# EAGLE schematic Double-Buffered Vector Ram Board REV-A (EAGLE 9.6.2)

## Sheet 1 of 4: Vector Ram Control
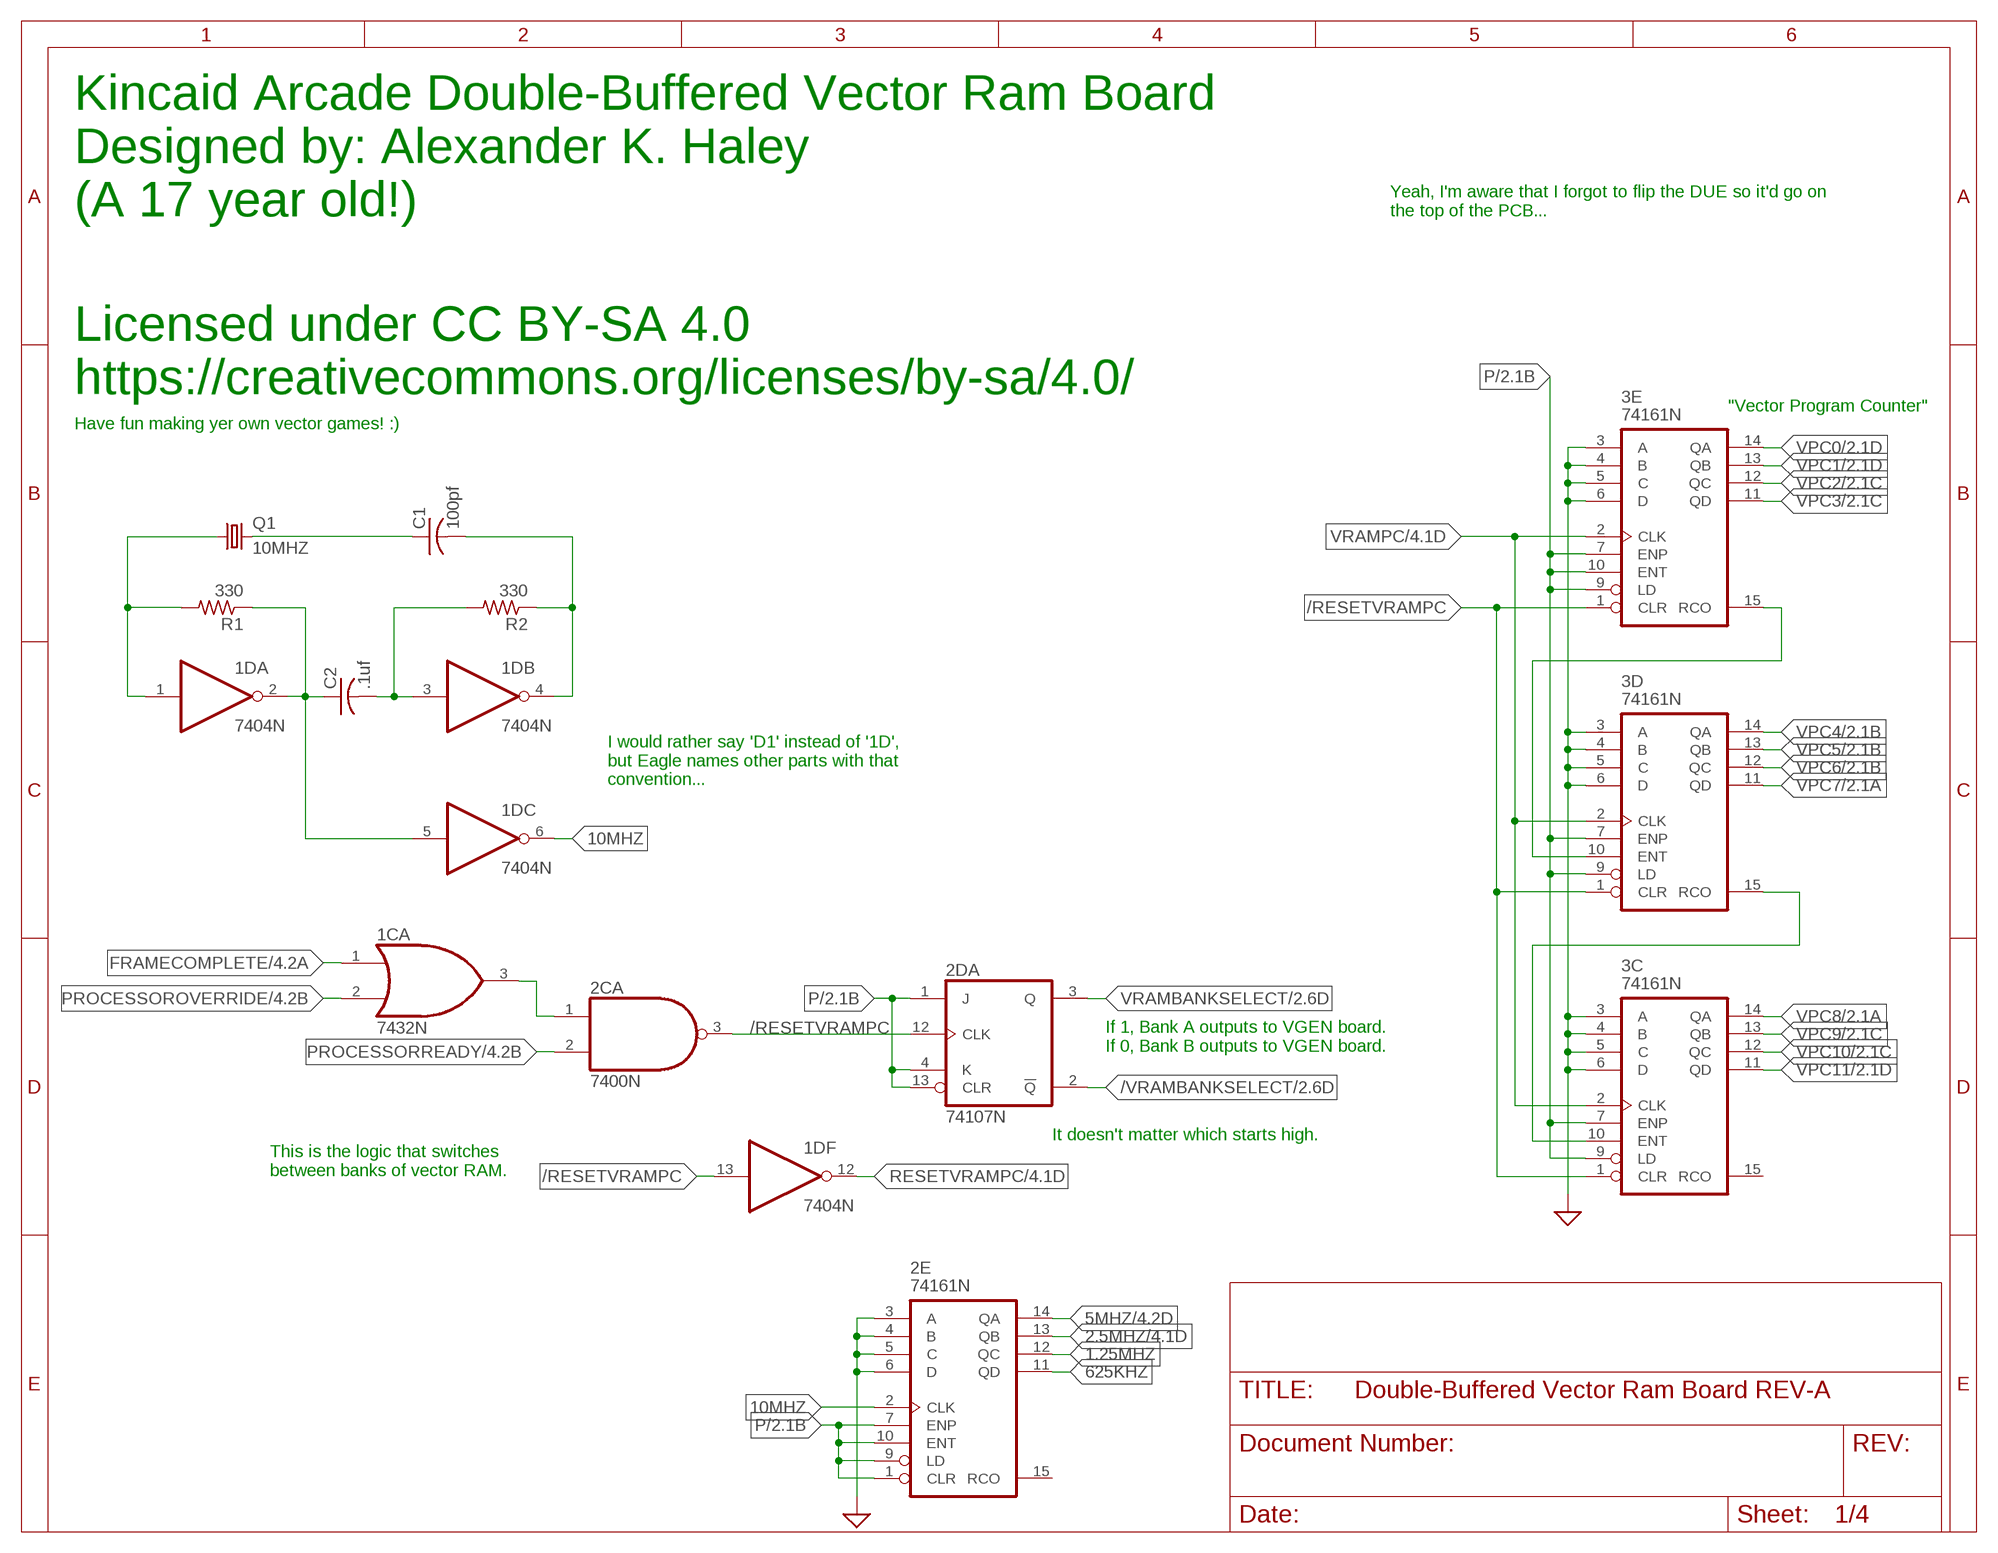
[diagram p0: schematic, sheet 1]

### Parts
1C  7432N  [DIL14]
1D  7404N  [DIL14]
2C  7400N  [DIL14]
2D  74107N  [DIL14]
2E  74161N  [DIL16]
3C  74161N  [DIL16]
3D  74161N  [DIL16]
3E  74161N  [DIL16]
C1  100pf  C-US025-030X050  [C025-030X050]
C2  .1uf  C-US050-050X075  [C050-050X075]
Q1  10MHZ  CRYSTALHC49S  [HC49/S]
R1  330  R-US_0207/10  [0207/10]
R2  330  R-US_0207/10  [0207/10]

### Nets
1.25MHZ: 2E.12(QC)
2.5MHZ: 2E.13(QB) ; also sheet 4
5MHZ: 2E.14(QA) ; also sheet 4
10MHZ: 1D.6(C:O) 2E.2(CLK)
625KHZ: 2E.11(QD)
/RESETVRAMPC: 1D.13(F:I) 2C.3(A:O) 2D.12(A:CLK) 3C.1(CLR) 3D.1(CLR) 3E.1(CLR)
/VRAMBANKSELECT: 2D.2(A:!Q) ; also sheet 2,3
FRAMECOMPLETE: 1C.1(A:I0) ; also sheet 4
GND: 2E.3(A) 2E.4(B) 2E.5(C) 2E.6(D) 3C.3(A) 3C.4(B) 3C.5(C) 3C.6(D) 3D.3(A) 3D.4(B) 3D.5(C) 3D.6(D) 3E.3(A) 3E.4(B) 3E.5(C) 3E.6(D) ; supply symbol labelled SUP ; also sheet 2,3,4
N$2: 1C.3(A:O) 2C.1(A:I0)
N$5: 3C.10(ENT) 3D.15(RCO)
N$6: 3D.10(ENT) 3E.15(RCO)
N$48: 1D.1(A:I) Q1.1 R1.2
N$52: 1D.2(A:O) 1D.5(C:I) C2.1 R1.1
N$61: 1D.3(B:I) C2.2 R2.2
N$69: C1.1 Q1.2
N$74: 1D.4(B:O) C1.2 R2.1
P: 2D.1(A:J) 2D.4(A:K) 2D.13(A:CLR) 2E.1(CLR) 2E.7(ENP) 2E.9(LD) 2E.10(ENT) 3C.7(ENP) 3C.9(LD) 3D.7(ENP) 3D.9(LD) 3E.7(ENP) 3E.9(LD) 3E.10(ENT) ; also sheet 2,3,4
PROCESSOROVERRIDE: 1C.2(A:I1) ; also sheet 4
PROCESSORREADY: 2C.2(A:I1) ; also sheet 4
RESETVRAMPC: 1D.12(F:O) ; also sheet 4
VPC0: 3E.14(QA) ; also sheet 2,3
VPC1: 3E.13(QB) ; also sheet 2,3
VPC2: 3E.12(QC) ; also sheet 2,3
VPC3: 3E.11(QD) ; also sheet 2,3
VPC4: 3D.14(QA) ; also sheet 2,3
VPC5: 3D.13(QB) ; also sheet 2,3
VPC6: 3D.12(QC) ; also sheet 2,3
VPC7: 3D.11(QD) ; also sheet 2,3
VPC8: 3C.14(QA) ; also sheet 2,3
VPC9: 3C.13(QB) ; also sheet 2,3
VPC10: 3C.12(QC) ; also sheet 2,3
VPC11: 3C.11(QD) ; also sheet 2,3
VRAMBANKSELECT: 2D.3(A:Q) ; also sheet 2,3
VRAMPC: 3C.2(CLK) 3D.2(CLK) 3E.2(CLK) ; also sheet 4
Unconnected: 2E.15(RCO) 3C.15(RCO)

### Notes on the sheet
- Kincaid Arcade Double-Buffered Vector Ram Board
- Designed by: Alexander K. Haley
- (A 17 year old!)
- Yeah, I'm aware that I forgot to flip the DUE so it'd go on
  the top of the PCB...
- Licensed under CC BY-SA 4.0
- https://creativecommons.org/licenses/by-sa/4.0/
- "Vector Program Counter"
- Have fun making yer own vector games! :)
- I would rather say 'D1' instead of '1D',
  but Eagle names other parts with that
  convention...
- If 1, Bank A outputs to VGEN board.
  If 0, Bank B outputs to VGEN board.
- It doesn't matter which starts high.
- This is the logic that switches 
  between banks of vector RAM.

## Sheet 2 of 4: Vector Ram Bank A
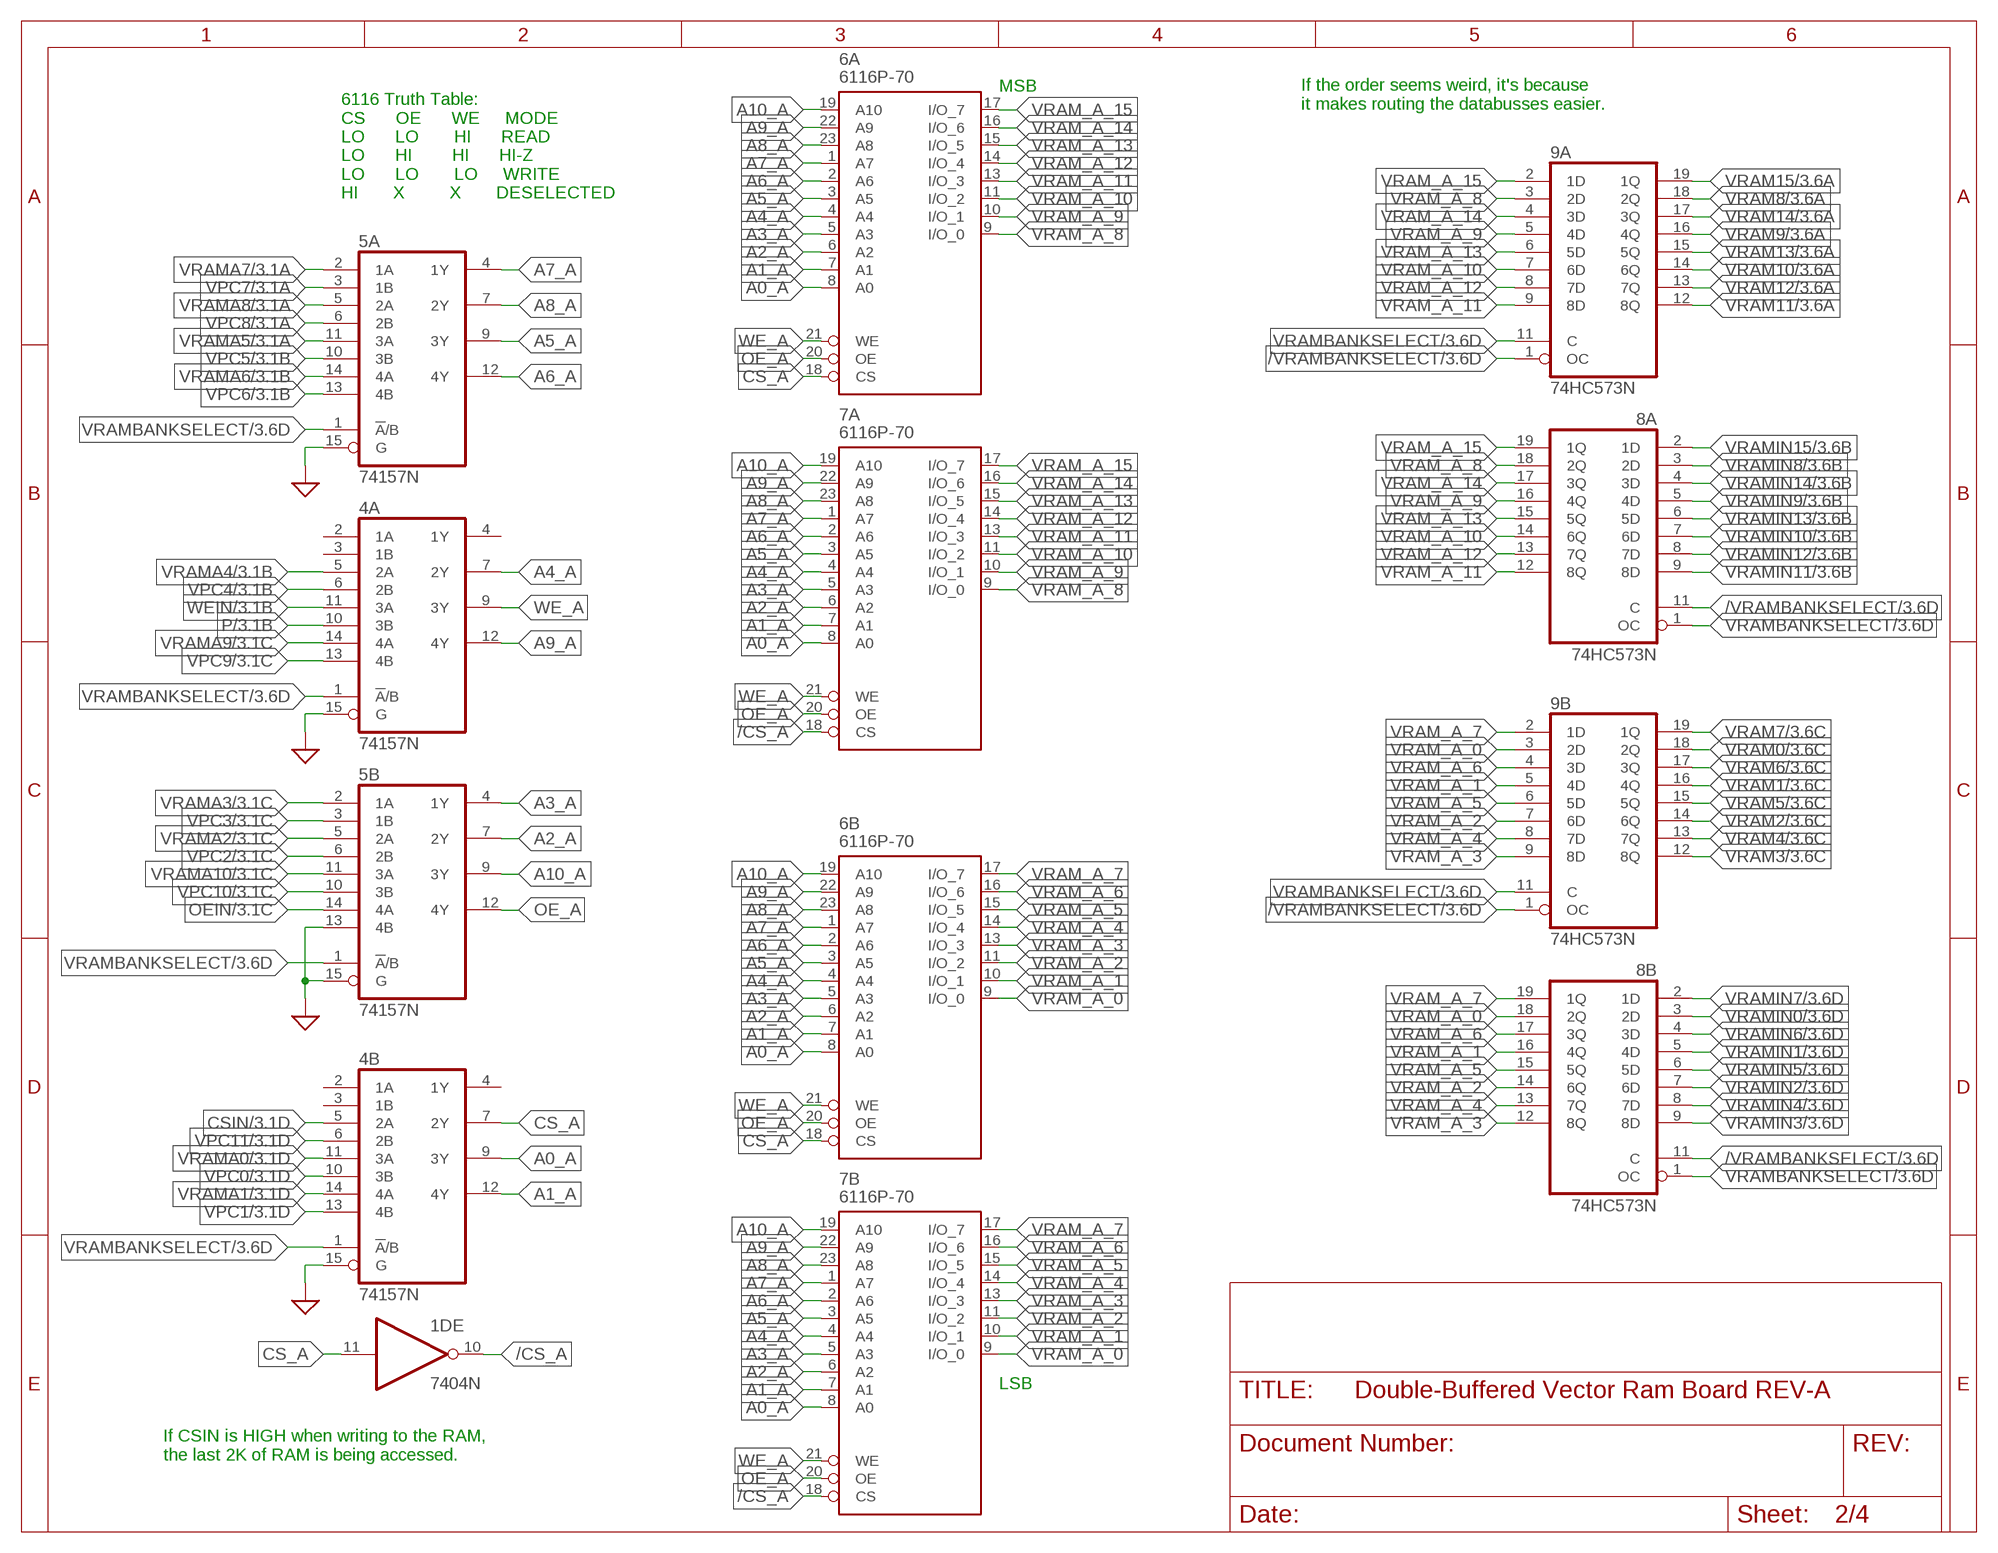
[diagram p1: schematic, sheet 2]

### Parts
4A  74157N  [DIL16]
4B  74157N  [DIL16]
5A  74157N  [DIL16]
5B  74157N  [DIL16]
6A  6116P-70  [DIL24]
6B  6116P-70  [DIL24]
7A  6116P-70  DS1220AB/AD  [DIL24]
7B  6116P-70  DS1220AB/AD  [DIL24]
8A  74HC573N  [DIL20]
8B  74HC573N  [DIL20]
9A  74HC573N  [DIL20]
9B  74HC573N  [DIL20]

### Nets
/CS_A: 1D.10(E:O) 7A.18(CS) 7B.18(CS)
/VRAMBANKSELECT: 8A.11(C) 8B.11(C) 9A.1(OC) 9B.1(OC) ; also sheet 1,3
A0_A: 4B.9(3Y) 6A.8(A0) 6B.8(A0) 7A.8(A0) 7B.8(A0)
A1_A: 4B.12(4Y) 6A.7(A1) 6B.7(A1) 7A.7(A1) 7B.7(A1)
A2_A: 5B.7(2Y) 6A.6(A2) 6B.6(A2) 7A.6(A2) 7B.6(A2)
A3_A: 5B.4(1Y) 6A.5(A3) 6B.5(A3) 7A.5(A3) 7B.5(A3)
A4_A: 4A.7(2Y) 6A.4(A4) 6B.4(A4) 7A.4(A4) 7B.4(A4)
A5_A: 5A.9(3Y) 6A.3(A5) 6B.3(A5) 7A.3(A5) 7B.3(A5)
A6_A: 5A.12(4Y) 6A.2(A6) 6B.2(A6) 7A.2(A6) 7B.2(A6)
A7_A: 5A.4(1Y) 6A.1(A7) 6B.1(A7) 7A.1(A7) 7B.1(A7)
A8_A: 5A.7(2Y) 6A.23(A8) 6B.23(A8) 7A.23(A8) 7B.23(A8)
A9_A: 4A.12(4Y) 6A.22(A9) 6B.22(A9) 7A.22(A9) 7B.22(A9)
A10_A: 5B.9(3Y) 6A.19(A10) 6B.19(A10) 7A.19(A10) 7B.19(A10)
CS_A: 1D.11(E:I) 4B.7(2Y) 6A.18(CS) 6B.18(CS)
CSIN: 4B.5(2A) ; also sheet 3,4
GND: 4A.15(G) 4B.15(G) 5A.15(G) 5B.13(4B) 5B.15(G) ; supply symbol labelled SUP ; also sheet 1,3,4
OE_A: 5B.12(4Y) 6A.20(OE) 6B.20(OE) 7A.20(OE) 7B.20(OE)
OEIN: 5B.14(4A) ; also sheet 3,4
P: 4A.10(3B) ; also sheet 1,3,4
VPC0: 4B.10(3B) ; also sheet 1,3
VPC1: 4B.13(4B) ; also sheet 1,3
VPC2: 5B.6(2B) ; also sheet 1,3
VPC3: 5B.3(1B) ; also sheet 1,3
VPC4: 4A.6(2B) ; also sheet 1,3
VPC5: 5A.10(3B) ; also sheet 1,3
VPC6: 5A.13(4B) ; also sheet 1,3
VPC7: 5A.3(1B) ; also sheet 1,3
VPC8: 5A.6(2B) ; also sheet 1,3
VPC9: 4A.13(4B) ; also sheet 1,3
VPC10: 5B.10(3B) ; also sheet 1,3
VPC11: 4B.6(2B) ; also sheet 1,3
VRAM0: 9B.18(2Q) ; also sheet 3,4
VRAM1: 9B.16(4Q) ; also sheet 3,4
VRAM2: 9B.14(6Q) ; also sheet 3,4
VRAM3: 9B.12(8Q) ; also sheet 3,4
VRAM4: 9B.13(7Q) ; also sheet 3,4
VRAM5: 9B.15(5Q) ; also sheet 3,4
VRAM6: 9B.17(3Q) ; also sheet 3,4
VRAM7: 9B.19(1Q) ; also sheet 3,4
VRAM8: 9A.18(2Q) ; also sheet 3,4
VRAM9: 9A.16(4Q) ; also sheet 3,4
VRAM10: 9A.14(6Q) ; also sheet 3,4
VRAM11: 9A.12(8Q) ; also sheet 3,4
VRAM12: 9A.13(7Q) ; also sheet 3,4
VRAM13: 9A.15(5Q) ; also sheet 3,4
VRAM14: 9A.17(3Q) ; also sheet 3,4
VRAM15: 9A.19(1Q) ; also sheet 3,4
VRAM_A_0: 6B.9(I/O_0) 7B.9(I/O_0) 8B.18(2Q) 9B.3(2D)
VRAM_A_1: 6B.10(I/O_1) 7B.10(I/O_1) 8B.16(4Q) 9B.5(4D)
VRAM_A_2: 6B.11(I/O_2) 7B.11(I/O_2) 8B.14(6Q) 9B.7(6D)
VRAM_A_3: 6B.13(I/O_3) 7B.13(I/O_3) 8B.12(8Q) 9B.9(8D)
VRAM_A_4: 6B.14(I/O_4) 7B.14(I/O_4) 8B.13(7Q) 9B.8(7D)
VRAM_A_5: 6B.15(I/O_5) 7B.15(I/O_5) 8B.15(5Q) 9B.6(5D)
VRAM_A_6: 6B.16(I/O_6) 7B.16(I/O_6) 8B.17(3Q) 9B.4(3D)
VRAM_A_7: 6B.17(I/O_7) 7B.17(I/O_7) 8B.19(1Q) 9B.2(1D)
VRAM_A_8: 6A.9(I/O_0) 7A.9(I/O_0) 8A.18(2Q) 9A.3(2D)
VRAM_A_9: 6A.10(I/O_1) 7A.10(I/O_1) 8A.16(4Q) 9A.5(4D)
VRAM_A_10: 6A.11(I/O_2) 7A.11(I/O_2) 8A.14(6Q) 9A.7(6D)
VRAM_A_11: 6A.13(I/O_3) 7A.13(I/O_3) 8A.12(8Q) 9A.9(8D)
VRAM_A_12: 6A.14(I/O_4) 7A.14(I/O_4) 8A.13(7Q) 9A.8(7D)
VRAM_A_13: 6A.15(I/O_5) 7A.15(I/O_5) 8A.15(5Q) 9A.6(5D)
VRAM_A_14: 6A.16(I/O_6) 7A.16(I/O_6) 8A.17(3Q) 9A.4(3D)
VRAM_A_15: 6A.17(I/O_7) 7A.17(I/O_7) 8A.19(1Q) 9A.2(1D)
VRAMA0: 4B.11(3A) ; also sheet 3,4
VRAMA1: 4B.14(4A) ; also sheet 3,4
VRAMA2: 5B.5(2A) ; also sheet 3,4
VRAMA3: 5B.2(1A) ; also sheet 3,4
VRAMA4: 4A.5(2A) ; also sheet 3,4
VRAMA5: 5A.11(3A) ; also sheet 3,4
VRAMA6: 5A.14(4A) ; also sheet 3,4
VRAMA7: 5A.2(1A) ; also sheet 3,4
VRAMA8: 5A.5(2A) ; also sheet 3,4
VRAMA9: 4A.14(4A) ; also sheet 3,4
VRAMA10: 5B.11(3A) ; also sheet 3,4
VRAMBANKSELECT: 4A.1(!A!/B) 4B.1(!A!/B) 5A.1(!A!/B) 5B.1(!A!/B) 8A.1(OC) 8B.1(OC) 9A.11(C) 9B.11(C) ; also sheet 1,3
VRAMIN0: 8B.3(2D) ; also sheet 3,4
VRAMIN1: 8B.5(4D) ; also sheet 3,4
VRAMIN2: 8B.7(6D) ; also sheet 3,4
VRAMIN3: 8B.9(8D) ; also sheet 3,4
VRAMIN4: 8B.8(7D) ; also sheet 3,4
VRAMIN5: 8B.6(5D) ; also sheet 3,4
VRAMIN6: 8B.4(3D) ; also sheet 3,4
VRAMIN7: 8B.2(1D) ; also sheet 3,4
VRAMIN8: 8A.3(2D) ; also sheet 3,4
VRAMIN9: 8A.5(4D) ; also sheet 3,4
VRAMIN10: 8A.7(6D) ; also sheet 3,4
VRAMIN11: 8A.9(8D) ; also sheet 3,4
VRAMIN12: 8A.8(7D) ; also sheet 3,4
VRAMIN13: 8A.6(5D) ; also sheet 3,4
VRAMIN14: 8A.4(3D) ; also sheet 3,4
VRAMIN15: 8A.2(1D) ; also sheet 3,4
WE_A: 4A.9(3Y) 6A.21(WE) 6B.21(WE) 7A.21(WE) 7B.21(WE)
WEIN: 4A.11(3A) ; also sheet 3,4
Unconnected: 4A.2(1A) 4A.3(1B) 4A.4(1Y) 4B.2(1A) 4B.3(1B) 4B.4(1Y)

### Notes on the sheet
- MSB
- If the order seems weird, it's because
  it makes routing the databusses easier.
- 6116 Truth Table:
  CS      OE      WE     MODE
  LO      LO       HI      READ
  LO      HI        HI      HI-Z
  LO      LO       LO     WRITE
  HI       X         X       DESELECTED
- LSB
- If CSIN is HIGH when writing to the RAM, 
  the last 2K of RAM is being accessed.

## Sheet 3 of 4: Vector Ram Bank B
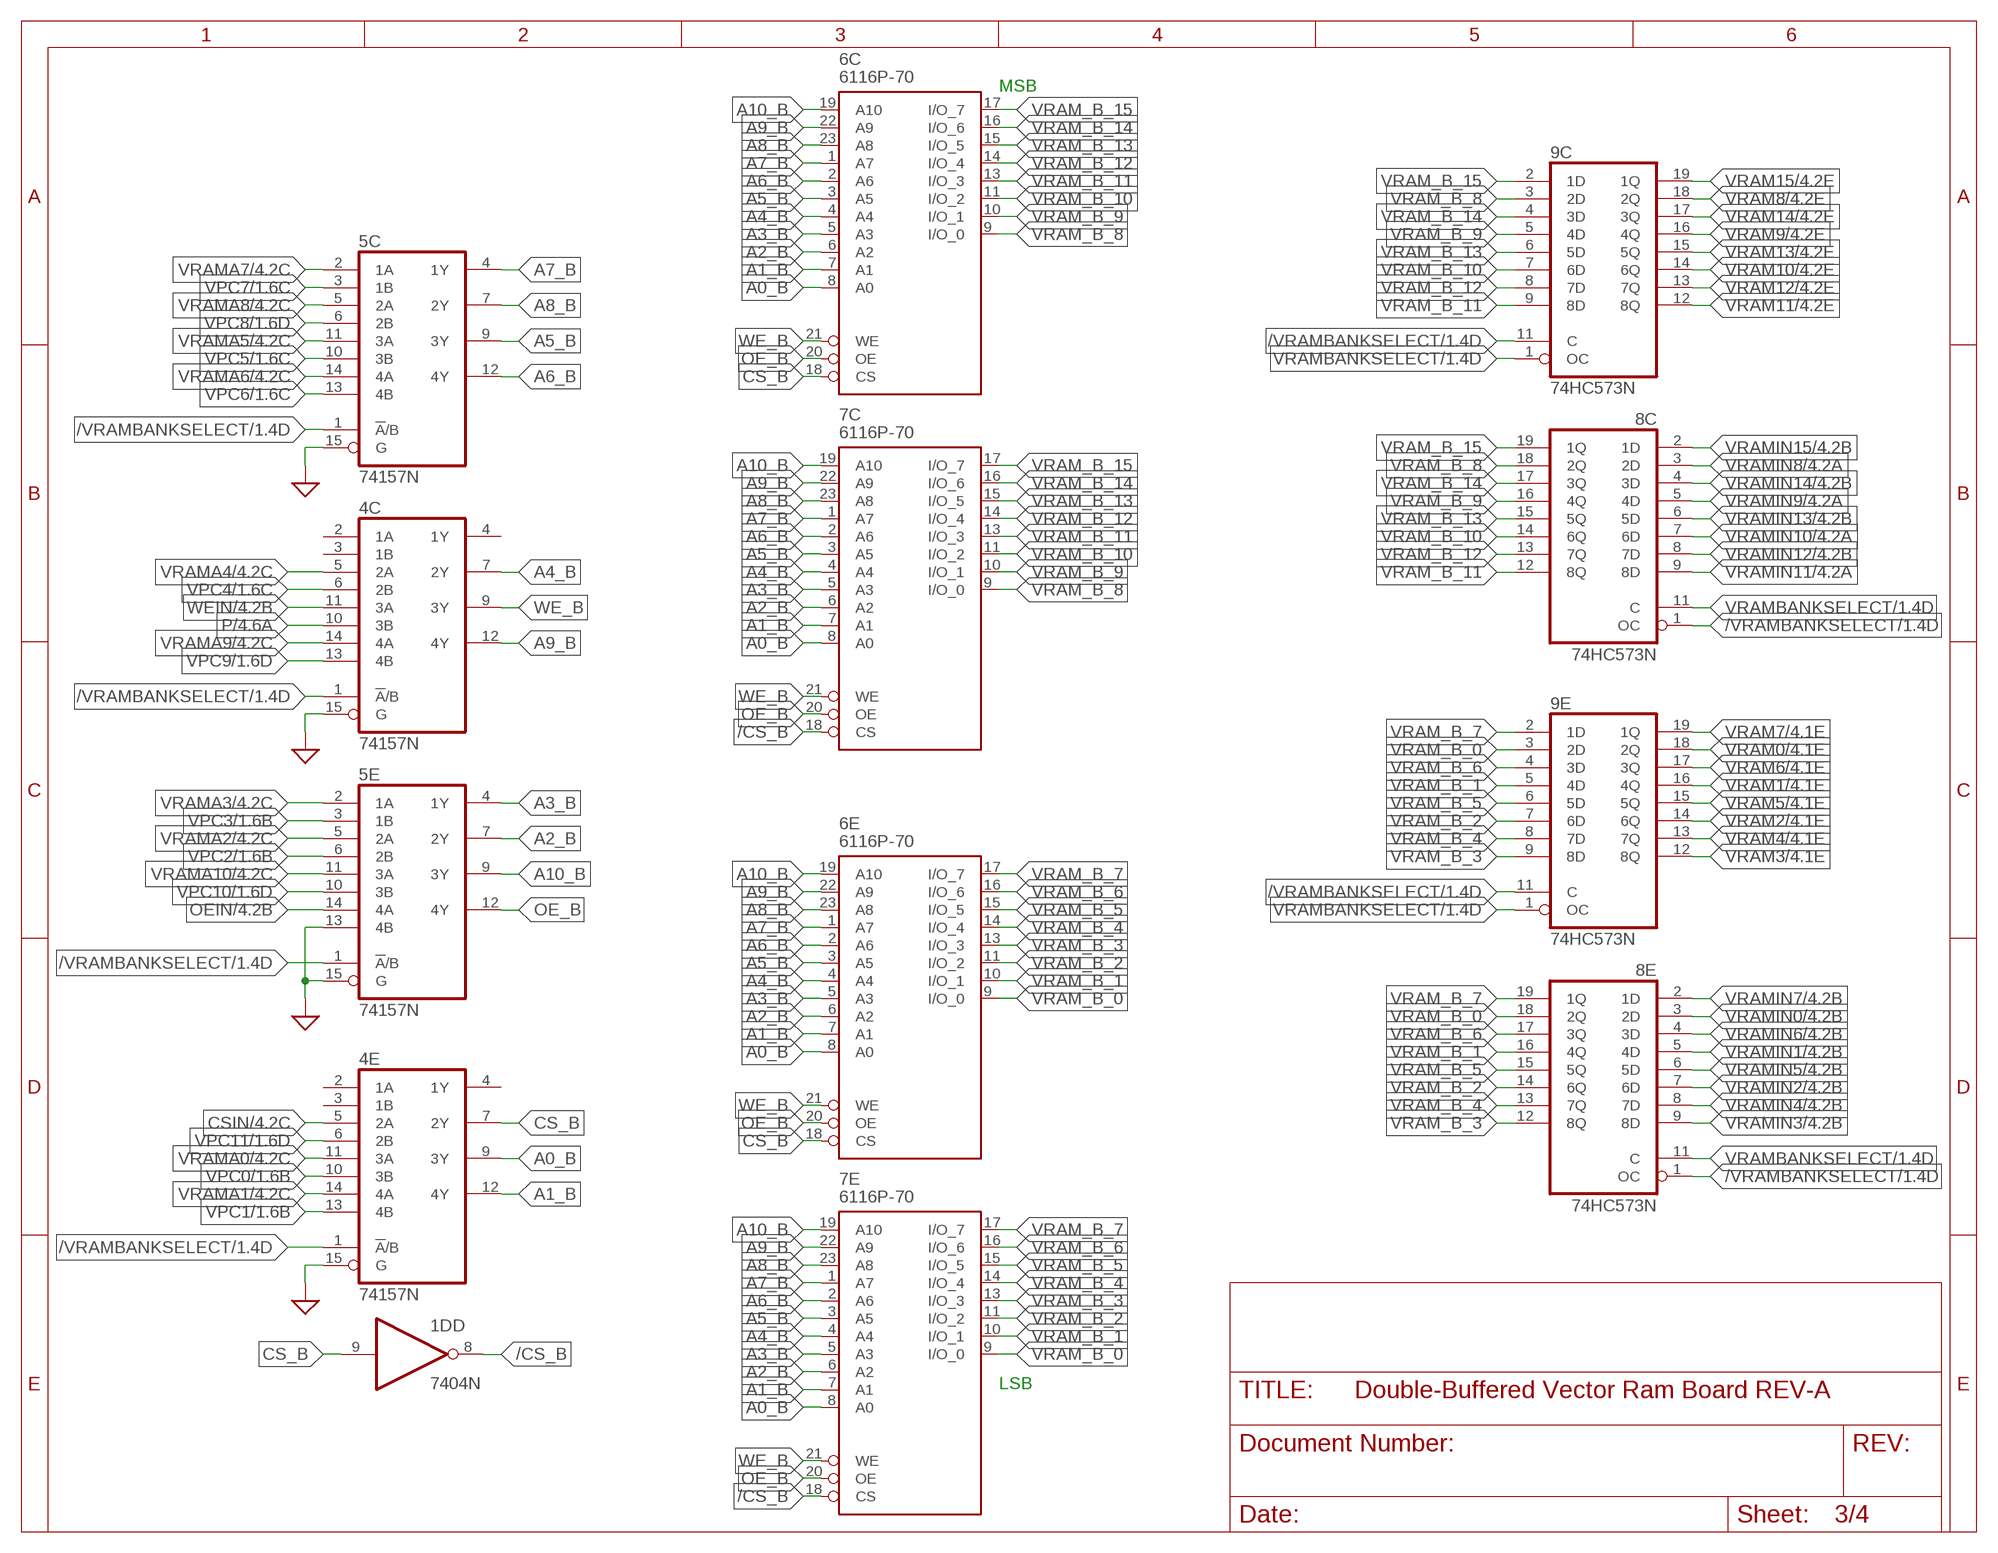
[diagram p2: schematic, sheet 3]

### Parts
4C  74157N  [DIL16]
4E  74157N  [DIL16]
5C  74157N  [DIL16]
5E  74157N  [DIL16]
6C  6116P-70  [DIL24]
6E  6116P-70  [DIL24]
7C  6116P-70  DS1220AB/AD  [DIL24]
7E  6116P-70  DS1220AB/AD  [DIL24]
8C  74HC573N  [DIL20]
8E  74HC573N  [DIL20]
9C  74HC573N  [DIL20]
9E  74HC573N  [DIL20]

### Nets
/CS_B: 1D.8(D:O) 7C.18(CS) 7E.18(CS)
/VRAMBANKSELECT: 4C.1(!A!/B) 4E.1(!A!/B) 5C.1(!A!/B) 5E.1(!A!/B) 8C.1(OC) 8E.1(OC) 9C.11(C) 9E.11(C) ; also sheet 1,2
A0_B: 4E.9(3Y) 6C.8(A0) 6E.8(A0) 7C.8(A0) 7E.8(A0)
A1_B: 4E.12(4Y) 6C.7(A1) 6E.7(A1) 7C.7(A1) 7E.7(A1)
A2_B: 5E.7(2Y) 6C.6(A2) 6E.6(A2) 7C.6(A2) 7E.6(A2)
A3_B: 5E.4(1Y) 6C.5(A3) 6E.5(A3) 7C.5(A3) 7E.5(A3)
A4_B: 4C.7(2Y) 6C.4(A4) 6E.4(A4) 7C.4(A4) 7E.4(A4)
A5_B: 5C.9(3Y) 6C.3(A5) 6E.3(A5) 7C.3(A5) 7E.3(A5)
A6_B: 5C.12(4Y) 6C.2(A6) 6E.2(A6) 7C.2(A6) 7E.2(A6)
A7_B: 5C.4(1Y) 6C.1(A7) 6E.1(A7) 7C.1(A7) 7E.1(A7)
A8_B: 5C.7(2Y) 6C.23(A8) 6E.23(A8) 7C.23(A8) 7E.23(A8)
A9_B: 4C.12(4Y) 6C.22(A9) 6E.22(A9) 7C.22(A9) 7E.22(A9)
A10_B: 5E.9(3Y) 6C.19(A10) 6E.19(A10) 7C.19(A10) 7E.19(A10)
CS_B: 1D.9(D:I) 4E.7(2Y) 6C.18(CS) 6E.18(CS)
CSIN: 4E.5(2A) ; also sheet 2,4
GND: 4C.15(G) 4E.15(G) 5C.15(G) 5E.13(4B) 5E.15(G) ; supply symbol labelled SUP ; also sheet 1,2,4
OE_B: 5E.12(4Y) 6C.20(OE) 6E.20(OE) 7C.20(OE) 7E.20(OE)
OEIN: 5E.14(4A) ; also sheet 2,4
P: 4C.10(3B) ; also sheet 1,2,4
VPC0: 4E.10(3B) ; also sheet 1,2
VPC1: 4E.13(4B) ; also sheet 1,2
VPC2: 5E.6(2B) ; also sheet 1,2
VPC3: 5E.3(1B) ; also sheet 1,2
VPC4: 4C.6(2B) ; also sheet 1,2
VPC5: 5C.10(3B) ; also sheet 1,2
VPC6: 5C.13(4B) ; also sheet 1,2
VPC7: 5C.3(1B) ; also sheet 1,2
VPC8: 5C.6(2B) ; also sheet 1,2
VPC9: 4C.13(4B) ; also sheet 1,2
VPC10: 5E.10(3B) ; also sheet 1,2
VPC11: 4E.6(2B) ; also sheet 1,2
VRAM0: 9E.18(2Q) ; also sheet 2,4
VRAM1: 9E.16(4Q) ; also sheet 2,4
VRAM2: 9E.14(6Q) ; also sheet 2,4
VRAM3: 9E.12(8Q) ; also sheet 2,4
VRAM4: 9E.13(7Q) ; also sheet 2,4
VRAM5: 9E.15(5Q) ; also sheet 2,4
VRAM6: 9E.17(3Q) ; also sheet 2,4
VRAM7: 9E.19(1Q) ; also sheet 2,4
VRAM8: 9C.18(2Q) ; also sheet 2,4
VRAM9: 9C.16(4Q) ; also sheet 2,4
VRAM10: 9C.14(6Q) ; also sheet 2,4
VRAM11: 9C.12(8Q) ; also sheet 2,4
VRAM12: 9C.13(7Q) ; also sheet 2,4
VRAM13: 9C.15(5Q) ; also sheet 2,4
VRAM14: 9C.17(3Q) ; also sheet 2,4
VRAM15: 9C.19(1Q) ; also sheet 2,4
VRAM_B_0: 6E.9(I/O_0) 7E.9(I/O_0) 8E.18(2Q) 9E.3(2D)
VRAM_B_1: 6E.10(I/O_1) 7E.10(I/O_1) 8E.16(4Q) 9E.5(4D)
VRAM_B_2: 6E.11(I/O_2) 7E.11(I/O_2) 8E.14(6Q) 9E.7(6D)
VRAM_B_3: 6E.13(I/O_3) 7E.13(I/O_3) 8E.12(8Q) 9E.9(8D)
VRAM_B_4: 6E.14(I/O_4) 7E.14(I/O_4) 8E.13(7Q) 9E.8(7D)
VRAM_B_5: 6E.15(I/O_5) 7E.15(I/O_5) 8E.15(5Q) 9E.6(5D)
VRAM_B_6: 6E.16(I/O_6) 7E.16(I/O_6) 8E.17(3Q) 9E.4(3D)
VRAM_B_7: 6E.17(I/O_7) 7E.17(I/O_7) 8E.19(1Q) 9E.2(1D)
VRAM_B_8: 6C.9(I/O_0) 7C.9(I/O_0) 8C.18(2Q) 9C.3(2D)
VRAM_B_9: 6C.10(I/O_1) 7C.10(I/O_1) 8C.16(4Q) 9C.5(4D)
VRAM_B_10: 6C.11(I/O_2) 7C.11(I/O_2) 8C.14(6Q) 9C.7(6D)
VRAM_B_11: 6C.13(I/O_3) 7C.13(I/O_3) 8C.12(8Q) 9C.9(8D)
VRAM_B_12: 6C.14(I/O_4) 7C.14(I/O_4) 8C.13(7Q) 9C.8(7D)
VRAM_B_13: 6C.15(I/O_5) 7C.15(I/O_5) 8C.15(5Q) 9C.6(5D)
VRAM_B_14: 6C.16(I/O_6) 7C.16(I/O_6) 8C.17(3Q) 9C.4(3D)
VRAM_B_15: 6C.17(I/O_7) 7C.17(I/O_7) 8C.19(1Q) 9C.2(1D)
VRAMA0: 4E.11(3A) ; also sheet 2,4
VRAMA1: 4E.14(4A) ; also sheet 2,4
VRAMA2: 5E.5(2A) ; also sheet 2,4
VRAMA3: 5E.2(1A) ; also sheet 2,4
VRAMA4: 4C.5(2A) ; also sheet 2,4
VRAMA5: 5C.11(3A) ; also sheet 2,4
VRAMA6: 5C.14(4A) ; also sheet 2,4
VRAMA7: 5C.2(1A) ; also sheet 2,4
VRAMA8: 5C.5(2A) ; also sheet 2,4
VRAMA9: 4C.14(4A) ; also sheet 2,4
VRAMA10: 5E.11(3A) ; also sheet 2,4
VRAMBANKSELECT: 8C.11(C) 8E.11(C) 9C.1(OC) 9E.1(OC) ; also sheet 1,2
VRAMIN0: 8E.3(2D) ; also sheet 2,4
VRAMIN1: 8E.5(4D) ; also sheet 2,4
VRAMIN2: 8E.7(6D) ; also sheet 2,4
VRAMIN3: 8E.9(8D) ; also sheet 2,4
VRAMIN4: 8E.8(7D) ; also sheet 2,4
VRAMIN5: 8E.6(5D) ; also sheet 2,4
VRAMIN6: 8E.4(3D) ; also sheet 2,4
VRAMIN7: 8E.2(1D) ; also sheet 2,4
VRAMIN8: 8C.3(2D) ; also sheet 2,4
VRAMIN9: 8C.5(4D) ; also sheet 2,4
VRAMIN10: 8C.7(6D) ; also sheet 2,4
VRAMIN11: 8C.9(8D) ; also sheet 2,4
VRAMIN12: 8C.8(7D) ; also sheet 2,4
VRAMIN13: 8C.6(5D) ; also sheet 2,4
VRAMIN14: 8C.4(3D) ; also sheet 2,4
VRAMIN15: 8C.2(1D) ; also sheet 2,4
WE_B: 4C.9(3Y) 6C.21(WE) 6E.21(WE) 7C.21(WE) 7E.21(WE)
WEIN: 4C.11(3A) ; also sheet 2,4
Unconnected: 4C.2(1A) 4C.3(1B) 4C.4(1Y) 4E.2(1A) 4E.3(1B) 4E.4(1Y)

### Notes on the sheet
- MSB
- LSB

## Sheet 4 of 4: Connectors, Pullups, and Filter Capacitors
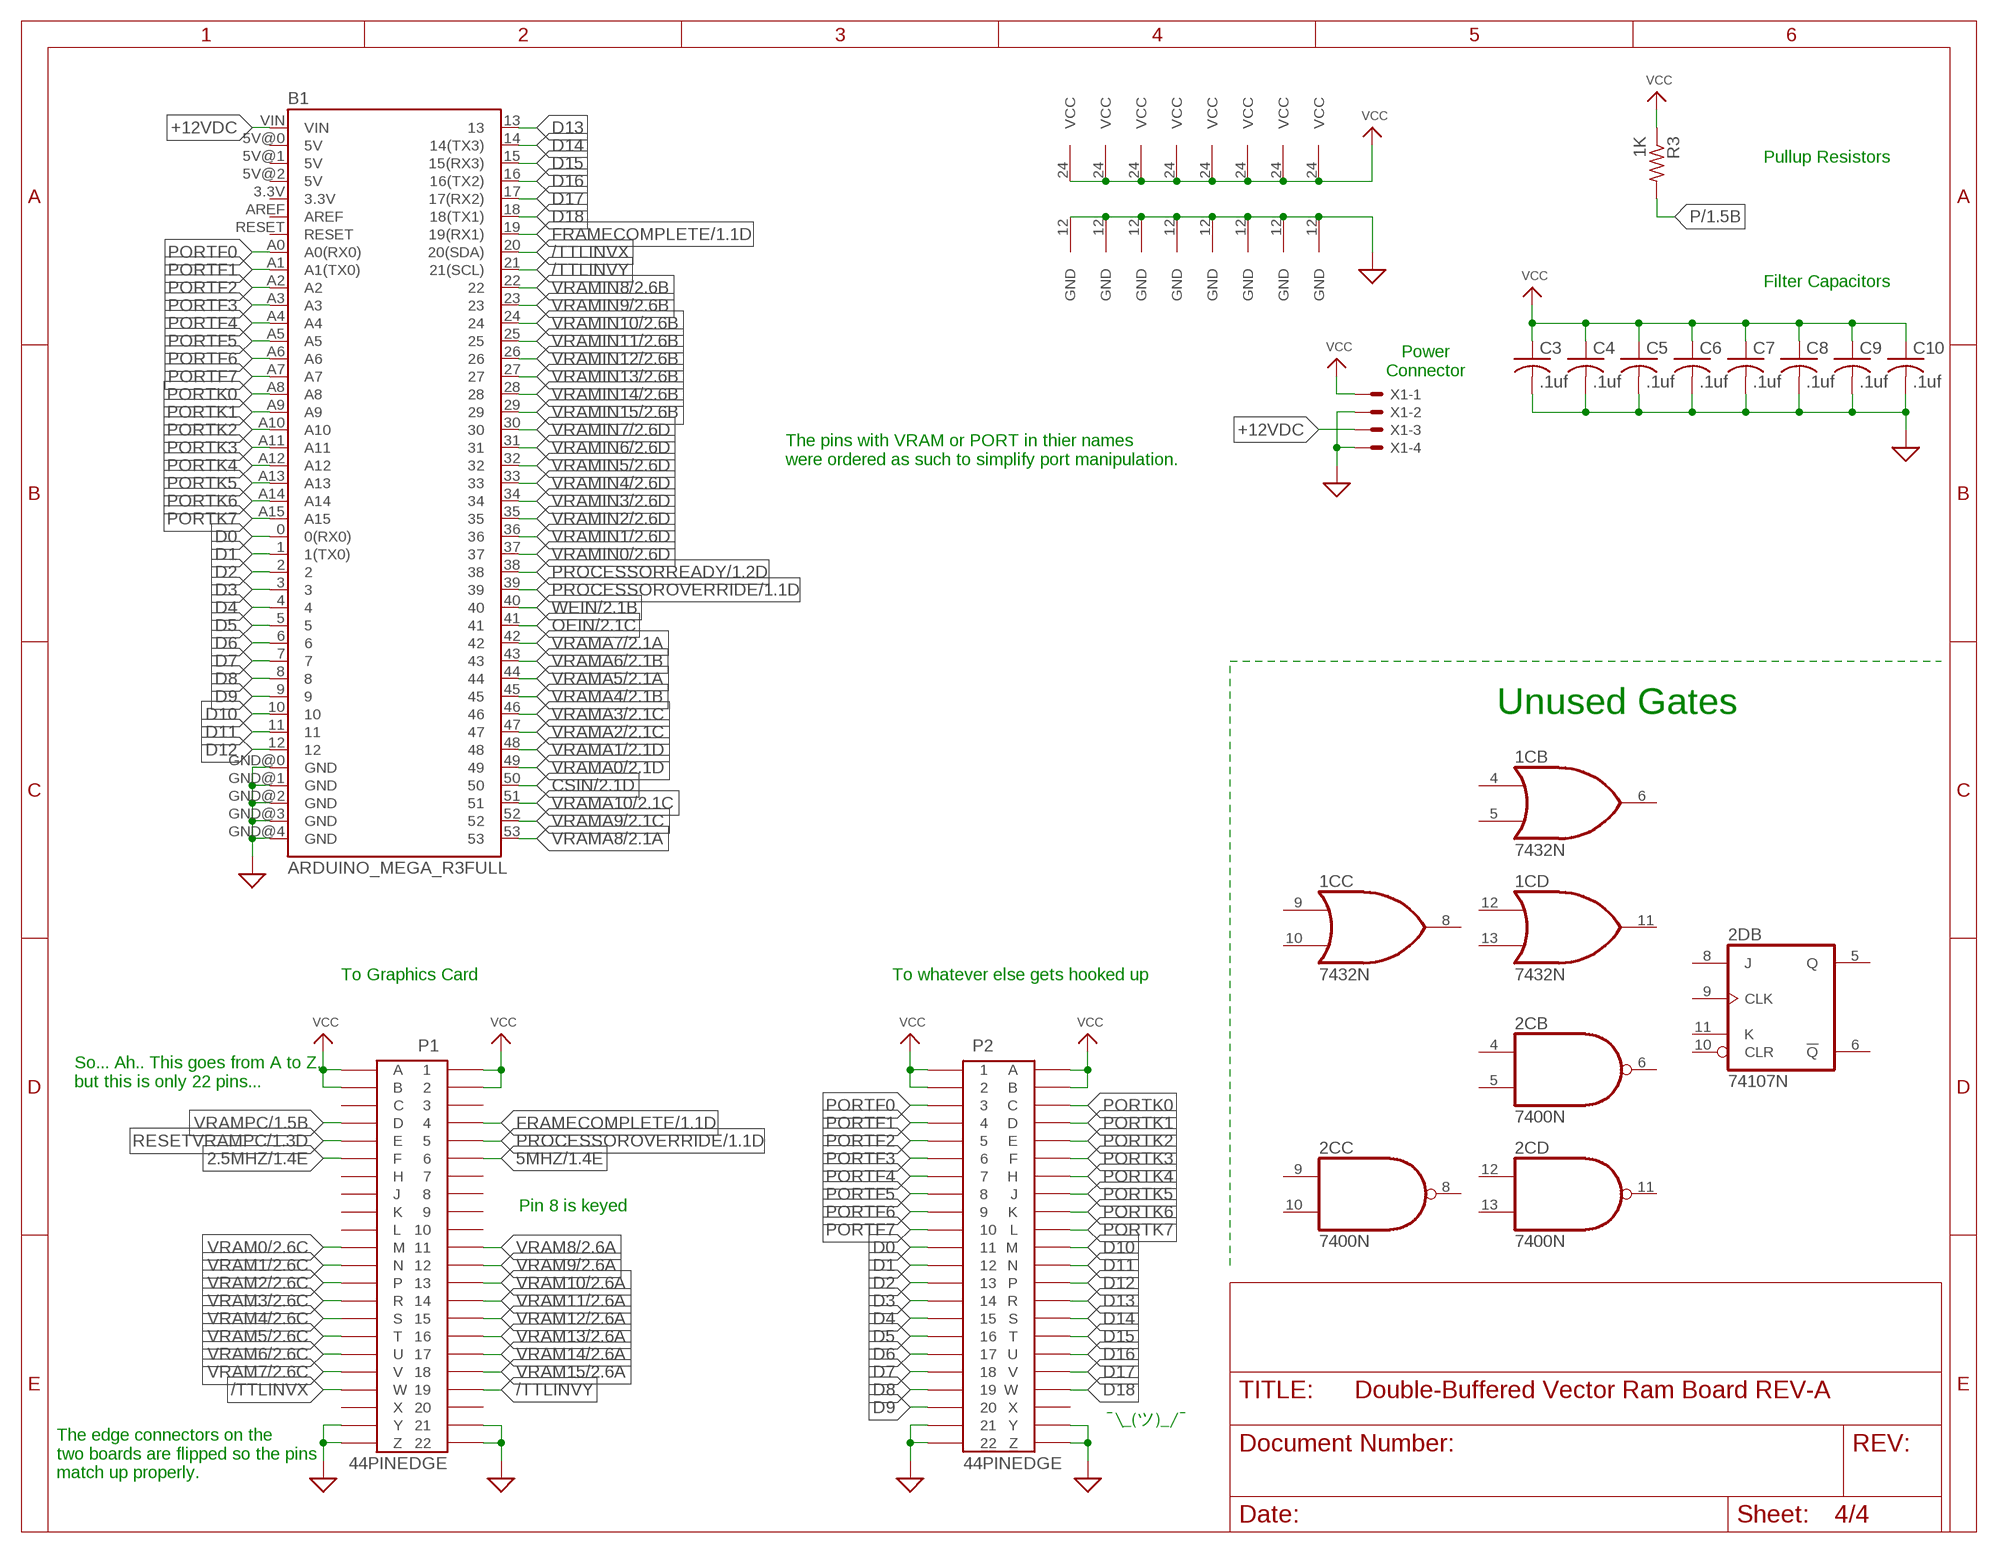
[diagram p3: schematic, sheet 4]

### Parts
B1  ARDUINO_MEGA_R3FULL  [ARDUINO_MEGA]
C3  .1uf  C-US050-025X075  [C050-025X075]
C4  .1uf  C-US050-025X075  [C050-025X075]
C5  .1uf  C-US050-025X075  [C050-025X075]
C6  .1uf  C-US050-025X075  [C050-025X075]
C7  .1uf  C-US050-025X075  [C050-025X075]
C8  .1uf  C-US050-025X075  [C050-025X075]
C9  .1uf  C-US050-025X075  [C050-025X075]
C10  .1uf  C-US050-025X075  [C050-025X075]
P1  44PINEDGE  [44PINEDGE]
P2  44PINEDGE  [44PINEDGE]
R3  1K  R-US_0207/12  [0207/12]
X1  KK-156-4  [KK-156-4]

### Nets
2.5MHZ: P1.F ; also sheet 1
5MHZ: P1.6 ; also sheet 1
+12VDC: B1.VIN X1.3
/TTLINVX: B1.20(20(SDA)) P1.W
/TTLINVY: B1.21(21(SCL)) P1.19
CSIN: B1.50 ; also sheet 2,3
D0: B1.0(0(RX0)) P2.11
D1: B1.1(1(TX0)) P2.12
D2: B1.2 P2.13
D3: B1.3 P2.14
D4: B1.4 P2.15
D5: B1.5 P2.16
D6: B1.6 P2.17
D7: B1.7 P2.18
D8: B1.8 P2.19
D9: B1.9 P2.20
D10: B1.10 P2.M
D11: B1.11 P2.N
D12: B1.12 P2.P
D13: B1.13 P2.R
D14: B1.14(14(TX3)) P2.S
D15: B1.15(15(RX3)) P2.T
D16: B1.16(16(TX2)) P2.U
D17: B1.17(17(RX2)) P2.V
D18: B1.18(18(TX1)) P2.W
FRAMECOMPLETE: B1.19(19(RX1)) P1.4 ; also sheet 1
GND: 6A.12(GND) 6B.12(GND) 6C.12(GND) 6E.12(GND) 7A.12(GND) 7B.12(GND) 7C.12(GND) 7E.12(GND) B1.GND@0(GND) B1.GND@1(GND) B1.GND@2(GND) B1.GND@3(GND) B1.GND@4(GND) C3.2 C4.2 C5.2 C6.2 C7.2 C8.2 C9.2 C10.2 P1.21 P1.22 P1.Y P1.Z P2.21 P2.22 P2.Y P2.Z X1.2 X1.4 ; supply symbol labelled SUP ; also sheet 1,2,3
OEIN: B1.41 ; also sheet 2,3
P: R3.2 ; also sheet 1,2,3
PORTF0: B1.A0(A0(RX0)) P2.3
PORTF1: B1.A1(A1(TX0)) P2.4
PORTF2: B1.A2 P2.5
PORTF3: B1.A3 P2.6
PORTF4: B1.A4 P2.7
PORTF5: B1.A5 P2.8
PORTF6: B1.A6 P2.9
PORTF7: B1.A7 P2.10
PORTK0: B1.A8 P2.C
PORTK1: B1.A9 P2.D
PORTK2: B1.A10 P2.E
PORTK3: B1.A11 P2.F
PORTK4: B1.A12 P2.H
PORTK5: B1.A13 P2.J
PORTK6: B1.A14 P2.K
PORTK7: B1.A15 P2.L
PROCESSOROVERRIDE: B1.39 P1.5 ; also sheet 1
PROCESSORREADY: B1.38 ; also sheet 1
RESETVRAMPC: P1.E ; also sheet 1
VCC: 6A.24(VCC) 6B.24(VCC) 6C.24(VCC) 6E.24(VCC) 7A.24(VCC) 7B.24(VCC) 7C.24(VCC) 7E.24(VCC) C3.1 C4.1 C5.1 C6.1 C7.1 C8.1 C9.1 C10.1 P1.1 P1.2 P1.A P1.B P2.1 P2.2 P2.A P2.B R3.1 X1.1
VRAM0: P1.M ; also sheet 2,3
VRAM1: P1.N ; also sheet 2,3
VRAM2: P1.P ; also sheet 2,3
VRAM3: P1.R ; also sheet 2,3
VRAM4: P1.S ; also sheet 2,3
VRAM5: P1.T ; also sheet 2,3
VRAM6: P1.U ; also sheet 2,3
VRAM7: P1.V ; also sheet 2,3
VRAM8: P1.11 ; also sheet 2,3
VRAM9: P1.12 ; also sheet 2,3
VRAM10: P1.13 ; also sheet 2,3
VRAM11: P1.14 ; also sheet 2,3
VRAM12: P1.15 ; also sheet 2,3
VRAM13: P1.16 ; also sheet 2,3
VRAM14: P1.17 ; also sheet 2,3
VRAM15: P1.18 ; also sheet 2,3
VRAMA0: B1.49 ; also sheet 2,3
VRAMA1: B1.48 ; also sheet 2,3
VRAMA2: B1.47 ; also sheet 2,3
VRAMA3: B1.46 ; also sheet 2,3
VRAMA4: B1.45 ; also sheet 2,3
VRAMA5: B1.44 ; also sheet 2,3
VRAMA6: B1.43 ; also sheet 2,3
VRAMA7: B1.42 ; also sheet 2,3
VRAMA8: B1.53 ; also sheet 2,3
VRAMA9: B1.52 ; also sheet 2,3
VRAMA10: B1.51 ; also sheet 2,3
VRAMIN0: B1.37 ; also sheet 2,3
VRAMIN1: B1.36 ; also sheet 2,3
VRAMIN2: B1.35 ; also sheet 2,3
VRAMIN3: B1.34 ; also sheet 2,3
VRAMIN4: B1.33 ; also sheet 2,3
VRAMIN5: B1.32 ; also sheet 2,3
VRAMIN6: B1.31 ; also sheet 2,3
VRAMIN7: B1.30 ; also sheet 2,3
VRAMIN8: B1.22 ; also sheet 2,3
VRAMIN9: B1.23 ; also sheet 2,3
VRAMIN10: B1.24 ; also sheet 2,3
VRAMIN11: B1.25 ; also sheet 2,3
VRAMIN12: B1.26 ; also sheet 2,3
VRAMIN13: B1.27 ; also sheet 2,3
VRAMIN14: B1.28 ; also sheet 2,3
VRAMIN15: B1.29 ; also sheet 2,3
VRAMPC: P1.D ; also sheet 1
WEIN: B1.40 ; also sheet 2,3
Unconnected: 1C.4(B:I0) 1C.5(B:I1) 1C.6(B:O) 1C.8(C:O) 1C.9(C:I0) 1C.10(C:I1) 1C.11(D:O) 1C.12(D:I0) 1C.13(D:I1) 2C.4(B:I0) 2C.5(B:I1) 2C.6(B:O) 2C.8(C:O) 2C.9(C:I0) 2C.10(C:I1) 2C.11(D:O) 2C.12(D:I0) 2C.13(D:I1) 2D.5(B:Q) 2D.6(B:!Q) 2D.8(B:J) 2D.9(B:CLK) 2D.10(B:CLR) 2D.11(B:K) B1.3.3V B1.5V@0(5V) B1.5V@1(5V) B1.5V@2(5V) B1.AREF B1.RESET P1.3 P1.7 P1.8 P1.9 P1.10 P1.20 P1.C P1.H P1.J P1.K P1.L P1.X P2.X

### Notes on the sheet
- Pullup Resistors
- Filter Capacitors
- Power
  Connector
- The pins with VRAM or PORT in thier names
  were ordered as such to simplify port manipulation.
- Unused Gates
- To Graphics Card | To whatever else gets hooked up
- So... Ah.. This goes from A to Z,
  but this is only 22 pins...
- Pin 8 is keyed
- ¯\_(ツ)_/¯
- The edge connectors on the
  two boards are flipped so the pins
  match up properly.

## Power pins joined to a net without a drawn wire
GND: 1C.7(P:GND) 1D.7(P:GND) 2C.7(P:GND) 2D.7(P:GND) 2E.8(GND) 3C.8(GND) 3D.8(GND) 3E.8(GND) 4A.8(GND) 4B.8(GND) 4C.8(GND) 4E.8(GND) 5A.8(GND) 5B.8(GND) 5C.8(GND) 5E.8(GND) 8A.10(GND) 8B.10(GND) 8C.10(GND) 8E.10(GND) 9A.10(GND) 9B.10(GND) 9C.10(GND) 9E.10(GND)
VCC: 1C.14(P:VCC) 1D.14(P:VCC) 2C.14(P:VCC) 2D.14(P:VCC) 2E.16(VCC) 3C.16(VCC) 3D.16(VCC) 3E.16(VCC) 4A.16(VCC) 4B.16(VCC) 4C.16(VCC) 4E.16(VCC) 5A.16(VCC) 5B.16(VCC) 5C.16(VCC) 5E.16(VCC) 8A.20(VCC) 8B.20(VCC) 8C.20(VCC) 8E.20(VCC) 9A.20(VCC) 9B.20(VCC) 9C.20(VCC) 9E.20(VCC)

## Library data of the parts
1C = 74xx-us:74*32: Quad 2-input OR gate
1D = 74xx-us:74*04: Hex INVERTER
2C = 74xx-us:74*00: Quad 2-input NAND gate
2D = 74xx-us:74*107: Dual J-K FLIP FLOP, clear
2E 3C 3D 3E = oldchips:74*161: Synchronous 4-bit COUNTER with direct clear
4A 4B 4C 4E 5A 5B 5C 5E = 74xx-us:74*157: Quadruple 2-line to 1-line data SELECTOR/MULTIPLEXER
6A 6B 6C 6E = OLD AND OBSOLETE ARCADE PARTS:6116P-70: 6116P-70, 16K SRAM
7A 7B 7C 7E = OLD AND OBSOLETE ARCADE PARTS:DS1220AB/AD: A nonvolatile SRAM chip, pin compatible with the 6116, 2716, or any other device that uses this standard.
8A 8B 8C 8E 9A 9B 9C 9E = 74xx-us:74*573: 8-bit D latch BUS DRIVER
B1 = SparkFun-Boards:ARDUINO_MEGA_R3: Arduino Mega R3 ATmega2560 R3 compatible footprint. SparkFun Products: Arduino Mega 2560 R3
C1-C10 = rcl:C-US: CAPACITOR, American symbol; SPICEPREFIX: C
P1 P2 = edge-156:44PINEDGE: 44 PIN EDGE CONNECTOR FOR PCB
Q1 = crystal:CRYSTAL: CRYSTAL; OC_FARNELL: 1667008; OC_NEWARK: unknown
R1 R2 = rcl:R-US_: RESISTOR, American symbol; SPICEPREFIX: R
R3 = resistor:R-US_: RESISTOR, American symbol
X1 = con-molex:KK-156-4: KK 156 HEADER Source: http://www.molex.com/pdm_docs/sd/026604100_sd.pdf; MF: MOLEX; OC_FARNELL: unknown; OC_NEWARK: unknown

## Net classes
0 default: width 0.381 mm, clearance 0.356 mm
